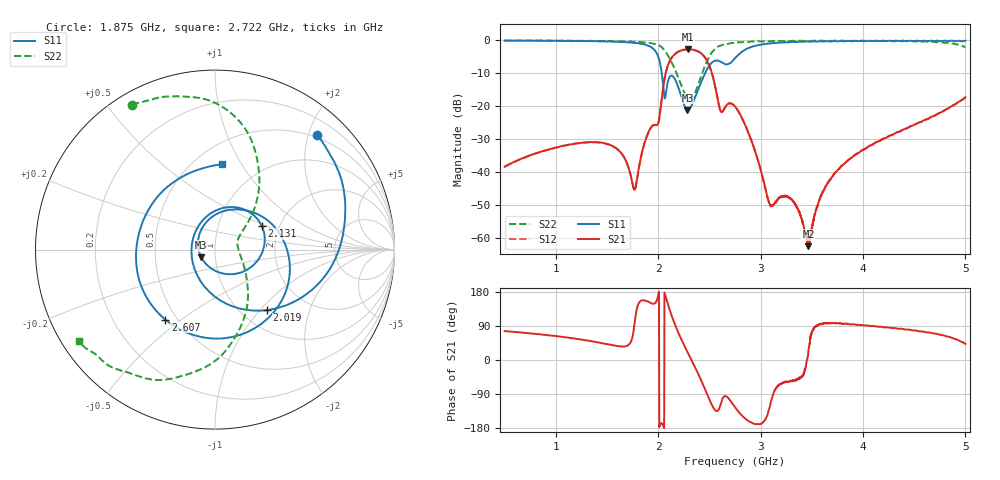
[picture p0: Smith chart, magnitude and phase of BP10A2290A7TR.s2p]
!Agilent Technologies,E8358A,US41080443,A.07.50.56
!Agilent E8358A: A.07.50.56
!Date: Tuesday, December 16, 2014 14:00:20
!Correction: S11(Full 2 Port(1,2))
!S21(Full 2 Port(1,2))
!S12(Full 2 Port(1,2))
!S22(Full 2 Port(1,2))
!S2P File: Measurements: S11, S21, S12, S22:
# Hz S  dB  R 50
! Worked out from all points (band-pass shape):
!   1601 points, 500 MHz to 5 GHz, reference 50 ohm
!   highest |S21| = -2.70 dB at 2.292 GHz (marker M1); lowest = -62.5 dB at 3.467 GHz (marker M2)
!   |S21| within 3 dB of the highest: 2.122 GHz to 2.469 GHz (346.3 MHz wide, 15.1 % of centre)
!   lowest |S11| = -21.2 dB at 2.286 GHz (marker M3), VSWR 1.19, Z = 42.7 - j3.61 ohm
!   |S11| at or under -10 dB: 2.035 GHz to 2.458 GHz (422.8 MHz wide, 18.8 % of centre)
!   |S22| runs from -17.9 to 0.0 dB; largest |S21 - S12| = 0.0041
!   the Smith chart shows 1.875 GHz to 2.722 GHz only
!   S11 on the Smith chart (normalised r, x): 1.875 GHz: 0.44, +2.15; 2.019 GHz: 1.30, -1.09; 2.131 GHz: 1.62, +0.47; 2.607 GHz: 0.43, -0.44; 2.722 GHz: 0.67, +0.83
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5e8  -0.08 163.7  -38.37 76.3  -38.38 76.4  -0.05 172.9
1.250938e9  -0.19 132.1  -31.08 53.9  -31.12 54.0  -0.12 157.3
1.599688e9  -0.39 103.2  -32.96 36.9  -33.00 37.0  -0.24 143.1
1.765625e9  -0.79 77.7  -45.33 89.2  -45.31 88.6  -0.44 131.3
1.875312e9  -1.33 48.4  -30.30 156.5  -30.29 156.8  -0.64 119.8
2.001875e9  -5.11 -28.2  -24.99 173.2  -24.98 173.4  -1.41 96.0
2.01875e9  -7.04 -49.3  -21.76 -170.0  -21.77 -170.2  -1.69 90.9
2.13125e9  -10.70 26.9  -5.27 117.0  -5.29 117.1  -6.66 57.8
2.285938e9  -21.16 -151.4  -2.71 20.9  -2.75 20.9  -17.40 21.0
2.291562e9  -21.15 -159.6  -2.70 17.9  -2.74 17.9  -17.56 18.6
2.435e9  -11.58 57.6  -4.37 -62.9  -4.39 -62.8  -9.49 -57.0
2.519375e9  -6.89 -26.8  -9.44 -115.8  -9.48 -115.8  -3.83 -92.9
2.606562e9  -6.41 -125.4  -21.29 -119.6  -21.32 -119.7  -1.60 -123.3
2.721875e9  -6.42 85.1  -19.29 -113.8  -19.29 -114.1  -0.79 -146.2
2.75e9  -5.40 55.9  -20.05 -124.7  -20.13 -124.4  -0.79 -149.6
2.854062e9  -2.73 -12.7  -25.97 -155.4  -26.00 -155.7  -0.41 -161.0
3.025625e9  -1.19 -65.9  -42.32 -163.7  -42.30 -163.5  -0.32 -172.2
3.467188e9  -0.38 -118.6  -62.47 27.8  -60.85 30.0  -0.12 170.2
3.500938e9  -0.31 -120.2  -57.71 72.8  -56.83 72.3  -0.17 170.0
3.720312e9  -0.20 -133.4  -40.52 97.5  -40.50 97.6  -0.07 165.1
4.251875e9  -0.09 -154.4  -29.07 85.6  -29.11 85.9  -0.22 153.7
5e9  -0.11 -175.7  -17.25 42.4  -17.29 42.5  -2.07 97.3
